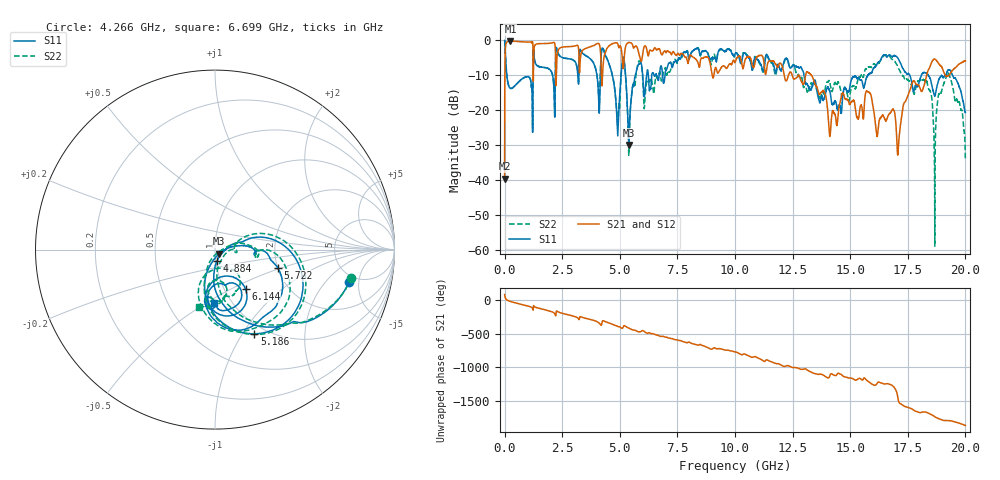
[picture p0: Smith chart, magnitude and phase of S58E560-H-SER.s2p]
!{S58E560}
!Johanson Technology Inc.
!www.johansontechnology.com
!Test Board Conditions:
!Substrate Type  RO4350B
!Substrate Thickness  60 mil
!Substrate Dk  3.66
!TL Type: GCPW
!TL Trace Width  115 mil
!TL Gap  52 mil
!Electrode orientation  Horizontal
!DUT TOPOLOGY	SERIES
!Mounting Pad LxW  55x428 mil
! Created Wed Apr 14 11:57:12 2021
# mhz S ma R 50
! 2 Port Network Data from SP1.SP block
! freq  magS11  angS11  magS21  angS21  magS12  angS12  magS22  angS22
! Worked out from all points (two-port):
!   20001 points, 300 kHz to 20 GHz, reference 50 ohm
!   highest |S21| = -0.20 dB at 251.3 MHz (marker M1); lowest = -39.6 dB at 300 kHz (marker M2)
!   |S21| within 3 dB of the highest: 27.81 MHz to 1.234 GHz (1.207 GHz wide, 191 % of centre); 1.268 GHz to 2.206 GHz (937.6 MHz wide, 54 % of centre)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
!   lowest |S11| = -30.0 dB at 5.391 GHz (marker M3), VSWR 1.07, Z = 52.1 - j2.44 ohm
!   |S11| at or under -10 dB: 96.4 MHz to 1.231 GHz (1.135 GHz wide, 171 % of centre); 13 GHz to 15.77 GHz (2.775 GHz wide, 19.3 % of centre); 18.39 GHz to 19.15 GHz (756 MHz wide, 4.03 % of centre)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
!   |S22| runs from -59.0 to 0.0 dB; largest |S21 - S12| = 0.0099
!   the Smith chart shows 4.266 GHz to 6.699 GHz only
!   S11 on the Smith chart (normalised r, x): 4.266 GHz: 4.23, -3.73; 4.884 GHz: 1.01, -0.13; 5.186 GHz: 0.88, -1.13; 5.722 GHz: 2.00, -0.47; 6.144 GHz: 1.25, -0.60; 6.699 GHz: 0.83, -0.54
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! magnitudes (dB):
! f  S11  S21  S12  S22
! 300 kHz  0.0  -39.6  -39.6  0.0
! 104.3 MHz  -10.5  -0.4  -0.4  -10.4
! 251.3 MHz  -13.7  -0.2  -0.2  -13.7
! 3.334 GHz  -3.2  -3.5  -3.5  -3.2
! 4.061 GHz  -13.7  -0.8  -0.8  -13.3
! 4.266 GHz  -2.3  -8.0  -7.9  -2.2
! 4.884 GHz  -23.9  -0.8  -0.7  -22.5
! 5.186 GHz  -5.7  -5.4  -5.4  -5.7
! 5.391 GHz  -30.0  -0.6  -0.6  -32.7
! 5.722 GHz  -8.8  -1.7  -1.7  -8.9
! 6.144 GHz  -11.1  -1.9  -1.9  -12.9
! 6.667 GHz  -11.4  -2.5  -2.5  -9.8
! 6.699 GHz  -10.6  -2.3  -2.3  -9.6
! 10 GHz  -3.9  -6.3  -6.3  -4.1
! 13.33 GHz  -13.5  -10.1  -10.0  -12.3
! 14.12 GHz  -14.6  -27.5  -27.4  -12.2
! 16.67 GHz  -4.2  -21.3  -21.1  -4.2
! 17.09 GHz  -5.3  -30.5  -30.4  -7.9
! 18.28 GHz  -9.3  -11.2  -11.2  -11.6
! 18.67 GHz  -15.8  -5.4  -5.3  -51.2
! 19.29 GHz  -8.4  -10.0  -10.0  -9.8
! 20 GHz  -20.6  -5.9  -5.8  -34.5
